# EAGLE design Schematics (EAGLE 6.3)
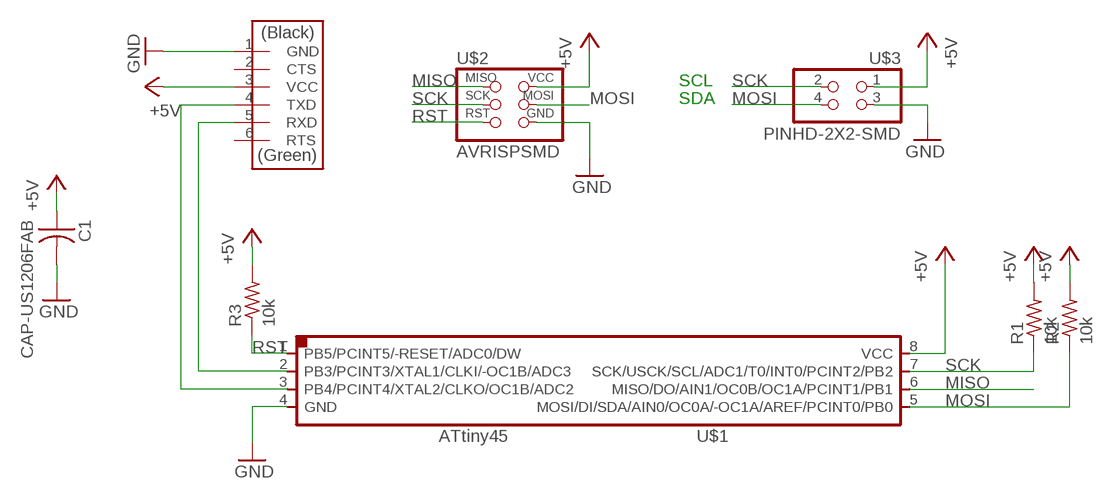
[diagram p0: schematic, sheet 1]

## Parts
C1  CAP-US1206FAB  [C1206FAB]
R1  10k  RES-US1206FAB  [R1206FAB]
R2  10k  RES-US1206FAB  [R1206FAB]
R3  10k  RES-US1206FAB  [R1206FAB]
U$1  ATTINY45SI  [SOIC8]
U$2  AVRISPSMD  [2X03SMD]
U$3  PINHD-2X2-SMD  [2X02SMD]
U$4  FTDI-SMD-HEADER  [1X06SMD]

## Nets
+5V: C1.1 R1.2 R2.2 R3.2 U$1.8(VCC) U$2.2(VCC) U$3.1 U$4.3(VCC)
GND: C1.2 U$1.4(GND) U$2.6(GND) U$3.3 U$4.1(GND)
MISO: U$1.6(MISO/DO/AIN1/OC0B/OC1A/PCINT1/PB1) U$2.1(MISO)
MOSI: R2.1 U$1.5(MOSI/DI/SDA/AIN0/OC0A/-OC1A/AREF/PCINT0/PB0) U$2.4(MOSI) U$3.4
N$1: U$1.3(PB4/PCINT4/XTAL2/CLKO/OC1B/ADC2) U$4.4(TXD)
N$2: U$1.2(PB3/PCINT3/XTAL1/CLKI/-OC1B/ADC3) U$4.5(RXD)
RST: R3.1 U$1.1(PB5/PCINT5/-RESET/ADC0/DW) U$2.5(RST)
SCK: R1.1 U$1.7(SCK/USCK/SCL/ADC1/T0/INT0/PCINT2/PB2) U$2.3(SCK) U$3.2
Unconnected: U$4.2(CTS) U$4.6(RTS)

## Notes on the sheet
- SCL
- SDA

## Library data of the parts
C1 = fab:CAP-US
R1-R3 = fab:RES-US: Resistor (US Symbol)
U$1 = fab:ATTINY45
U$2 = fab:AVRISP
U$3 = fab:PINHD-2X2-SMD
U$4 = fab:FTDI-SMD-HEADER

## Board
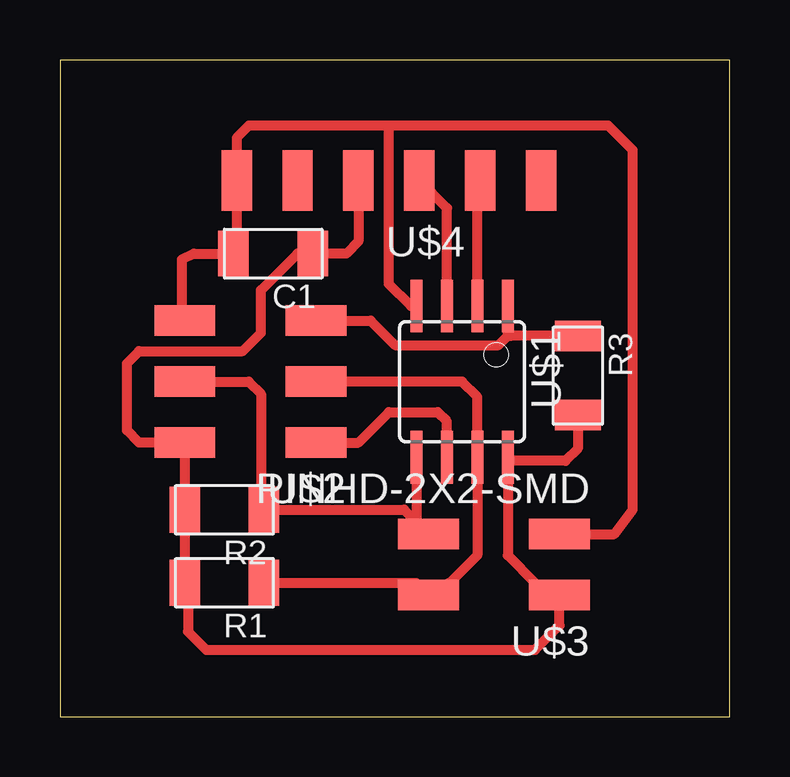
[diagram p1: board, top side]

Size 27.94 x 27.37 mm. Coordinates in mm from the lower left corner, seen from the top.
Outline: 0,0 27.94,0 27.94,27.37 0,27.37 0,0
Copper layers (1*16): Top 0.035mm / dielectric 1.5mm / Bottom 0.035mm
Design rules "default": minimum track width 10mil, minimum drill 24mil, track to track 8mil, track to pad 8mil, pad to pad 8mil, via to via 8mil, smd to smd 8mil, copper to edge 40mil, drill to drill 8mil, minimum pad ring 10mil, minimum via ring 8mil, stop-mask expansion 4mil, vias tented up to drill 0mil, thermal gap 10mil

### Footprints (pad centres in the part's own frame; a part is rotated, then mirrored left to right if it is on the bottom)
C1206FAB = smd 1.27 x 1.905: 1 -1.651,0; 2 1.651,0
R1206FAB = smd 1.27 x 1.905: 1 -1.651,0; 2 1.651,0
SOIC8 = smd 0.5 x 2.2: 1 -1.905,-3.154; 2 -0.645,-3.154; 3 0.625,-3.154; 4 1.895,-3.154; 5 1.905,3.154; 6 0.635,3.154; 7 -0.635,3.154; 8 -1.905,3.154
2X03SMD = smd 2.54 x 1.27: 1 -2.54,2.54; 2 2.92,2.54; 3 -2.54,0; 4 2.92,0; 5 -2.54,-2.54; 6 2.92,-2.54
2X02SMD = smd 2.54 x 1.27: 1 -2.54,1.27; 2 2.92,1.27; 3 -2.54,-1.27; 4 2.92,-1.27
1X06SMD = smd 2.54 x 1.27: 1 0,6.35; 2 0,3.81; 3 0,1.27; 4 0,-1.27; 5 0,-3.81; 6 0,-6.35

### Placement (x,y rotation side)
C1  8.89,19.3 180 top
R1  6.86,5.59 180 top
R2  6.86,8.64 180 top
R3  21.59,14.22 270 top
U$1  16.76,13.97 180 top
U$2  8.13,13.97 180 top
U$3  18.29,6.35 180 top
U$4  13.72,22.35 90 top

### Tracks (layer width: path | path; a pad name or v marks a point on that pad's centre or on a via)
+5V
  Top 0.406: U$2.2 R1.2 | U$2.2 5.21,5.46 5.08,5.33 | U$2.2 R2.2 | U$2.2 5.21,5.46 5.33,5.33 5.33,3.56 6.1,2.79 19.81,2.79 20.83,3.81 U$3.1 20.57,4.83 20.07,4.83 19.81,5.08 19.81,5.59 18.67,6.73 U$1.8 18.82,10.67 21.08,10.67 21.59,11.18 R3.2 | U$4.3 12.45,19.81 11.94,19.3 C1.1 9.91,19.3 8.38,17.78 8.38,16 7.62,15.24 3.3,15.24 2.79,14.73 2.79,11.94 3.3,11.43 U$2.2
GND
  Top 0.406: U$2.6 5.08,16.64 5.08,19.05 5.59,19.3 C1.2 7.37,19.43 U$4.1 7.62,22.61 7.62,22.86 7.37,23.11 7.37,24.13 7.87,24.64 13.72,24.64 | U$3.3 23.11,7.62 23.88,8.64 23.88,23.62 22.86,24.64 13.72,24.64 | U$1.4 14.63,17.12 13.72,18.03 13.72,24.64
MISO
  Top 0.406: U$2.1 12.45,11.43 13.72,12.7 15.75,12.7 16.13,12.32 U$1.6
MOSI
  Top 0.406: U$1.5 14.86,8.13 U$3.4 14.35,8.64 R2.1 8.38,8.76 8.38,13.46 7.87,13.97 U$2.4
N$1
  Top 0.406: U$1.3 16.14,21.2 U$4.4
N$2
  Top 0.406: U$1.2 17.41,22.23 U$4.5
RST
  Top 0.406: U$2.5 12.95,16.51 13.97,15.49 18.29,15.49 18.67,15.88 18.67,16 | U$1.1 18.67,16 | R3.1 18.8,15.88 18.67,16
SCK
  Top 0.406: R1.1 14.86,5.59 U$3.2 16.26,5.59 17.4,6.73 U$1.7 17.4,13.34 16.76,13.97 U$2.3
